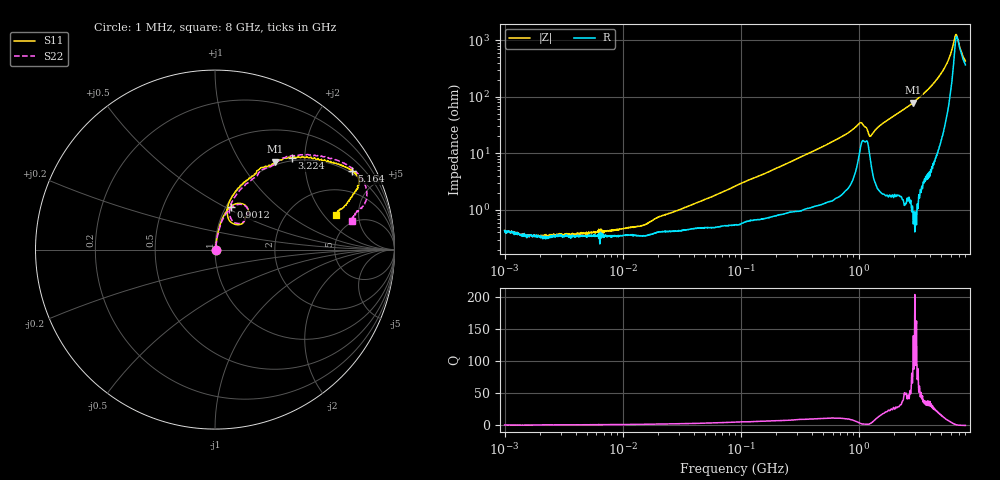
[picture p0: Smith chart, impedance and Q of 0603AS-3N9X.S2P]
!s-Parameter Generated by FASTRON Sdn. Bhd.
!FASTRON P/N : 0603AS-3N9X
!Keysight Technologies: E5071C_MY46733604_B.14.02
!Date: Tue Oct 24 10:31:39 2023
!Version  :Rev01  Tue Oct 24 10:31:39 2023
!Data & Calibration Information:
!Freq  S11:SOLT2(ON)  S21:SOLT2(ON)  S12:SOLT2(ON)  S22:SOLT2(ON)
!PortZ  Port1:50+j0  Port2:50+j0
!When reading reference impedance value at option line is always used.
! Remarks : This data is being provided solely for informational purposes.
# Hz S dB R 50
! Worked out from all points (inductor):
!   1601 points, 1 MHz to 8 GHz, reference 50 ohm
!   read as one part in series: L = 4.59 nH near 49.32 MHz
!   highest Q = 88.5 at 2.898 GHz (marker M1), where L = 4.35 nH
!   self-resonance near 6.895 GHz
!   S11 on the Smith chart (normalised r, x): 1 MHz: 1.01, -0.00; 901.2 MHz: 1.05, +0.54; 3.224 GHz: 0.94, +1.74; 5.164 GHz: 0.90, +3.53; 8 GHz: 3.57, +2.72
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1000000  -46.64 -2.7  -0.03 -0.1  -0.04 0.0  -46.75 2.7
1541011  -51.30 -12.3  -0.03 -0.1  -0.03 -0.0  -47.14 -23.1
2311589  -49.57 17.2  -0.04 -0.1  -0.04 -0.1  -53.64 32.8
2905262  -50.08 15.7  -0.04 -0.1  -0.04 -0.1  -50.90 13.5
4479405  -48.73 25.4  -0.03 -0.1  -0.04 -0.1  -50.34 31.2
8407329  -47.62 35.2  -0.03 -0.2  -0.03 -0.2  -48.01 37.7
1.449233e7  -53.24 52.3  -0.03 -0.3  -0.04 -0.3  -44.31 39.0
1.552719e7  -52.61 58.3  -0.03 -0.3  -0.04 -0.3  -43.95 41.4
2.00676e7  -43.32 57.7  -0.03 -0.4  -0.04 -0.3  -42.21 61.1
8.994653e7  -31.71 78.1  -0.05 -1.5  -0.06 -1.5  -31.99 76.7
4.006501e8  -19.53 79.8  -0.16 -5.9  -0.17 -5.9  -19.52 79.0
9.011973e8  -11.91 70.1  -0.65 -14.3  -0.66 -14.4  -11.90 68.5
1.035959e9  -10.51 54.4  -1.48 -15.8  -1.49 -15.8  -10.64 52.8
1.256741e9  -14.87 63.6  -0.83 -9.6  -0.84 -9.7  -14.51 59.8
1.7949e9  -8.73 69.4  -0.93 -21.4  -0.94 -21.5  -8.76 67.0
2.89772e9  -4.53 55.5  -2.81 -37.8  -2.83 -37.8  -4.66 55.2
3.223742e9  -3.51 50.0  -3.61 -40.6  -3.62 -40.7  -3.55 51.3
4.075033e9  -1.99 38.2  -6.01 -50.1  -6.00 -50.1  -1.94 40.3
5.164399e9  -1.11 29.9  -10.68 -56.4  -10.67 -56.4  -1.00 30.2
5.696244e9  -0.96 27.7  -13.91 -56.2  -13.91 -56.3  -0.85 26.1
6.65058e9  -1.38 23.0  -23.48 -11.8  -23.47 -12.1  -1.09 17.8
8e9  -3.05 15.9  -15.20 42.6  -15.20 42.2  -2.14 11.9
